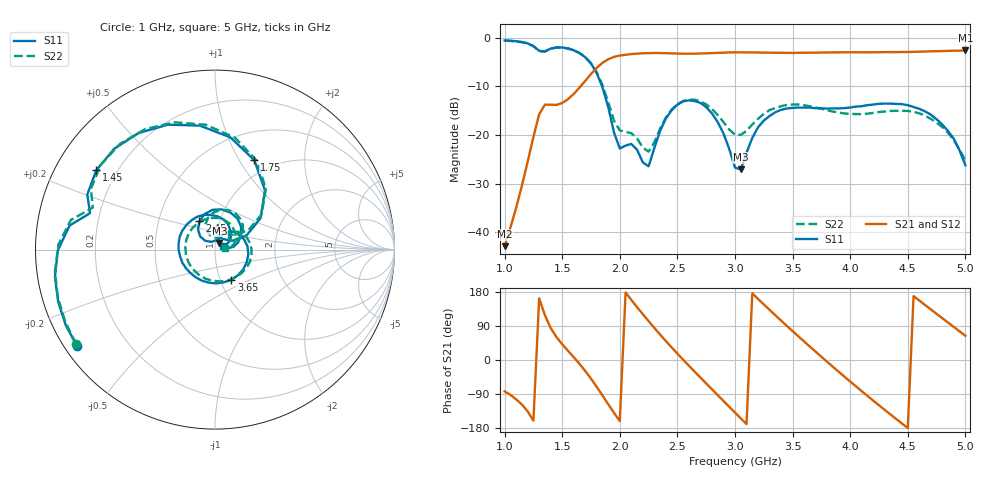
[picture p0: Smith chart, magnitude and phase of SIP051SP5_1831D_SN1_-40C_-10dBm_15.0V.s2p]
# GHz  S  dB  R  50
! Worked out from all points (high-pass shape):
!   81 points, 1 GHz to 5 GHz, reference 50 ohm
!   highest |S21| = -2.62 dB at 5 GHz (marker M1); lowest = -42.8 dB at 1 GHz (marker M2)
!   |S21| within 3 dB of the highest: 1.827 GHz to end of sweep
!   lowest |S11| = -27.1 dB at 3.05 GHz (marker M3), VSWR 1.09, Z = 52.4 + j3.84 ohm
!   |S11| at or under -10 dB: 1.846 GHz to end of sweep
!   |S22| runs from -25.2 to -0.6 dB; largest |S21 - S12| = 0.0022
!   S11 on the Smith chart (normalised r, x): 1 GHz: 0.03, -0.31; 1.45 GHz: 0.12, +0.30; 1.75 GHz: 0.82, +1.16; 2.45 GHz: 0.80, +0.26; 3.65 GHz: 1.13, -0.39; 5 GHz: 1.09, +0.05
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1  -0.55 -145.0  -42.85 -82.8  -43.25 -83.3  -0.58 -145.8
1.3  -2.68 164.6  -15.73 162.6  -15.70 162.4  -2.73 162.0
1.45  -1.99 146.2  -13.80 60.6  -13.80 60.5  -2.02 143.3
1.7  -4.00 82.1  -8.86 -28.9  -8.86 -28.9  -3.97 79.9
1.75  -5.29 66.2  -7.45 -49.3  -7.44 -49.3  -5.24 64.8
1.9  -14.29 24.2  -4.42 -116.9  -4.41 -116.8  -13.28 30.3
2.05  -22.17 74.4  -3.50 178.2  -3.49 178.4  -19.35 60.5
2.25  -26.43 115.5  -3.16 102.6  -3.15 102.6  -23.41 89.7
2.35  -19.11 138.5  -3.14 67.1  -3.13 67.1  -18.66 114.3
2.45  -14.90 119.0  -3.21 33.3  -3.20 33.2  -14.76 101.8
2.75  -14.26 41.5  -3.20 -61.9  -3.19 -61.8  -13.70 41.1
3  -26.70 21.0  -3.00 -138.9  -2.99 -138.8  -19.92 30.8
3.05  -27.08 55.7  -2.99 -153.9  -2.99 -154.0  -19.98 39.7
3.2  -18.40 56.1  -3.03 161.2  -3.03 161.2  -16.68 42.5
3.4  -14.81 6.0  -3.09 104.0  -3.08 103.9  -14.06 10.6
3.65  -14.36 -61.5  -3.06 35.3  -3.06 35.3  -14.08 -42.2
3.7  -14.47 -74.8  -3.06 21.9  -3.05 21.9  -14.35 -54.8
4.05  -14.15 -158.2  -2.98 -69.5  -2.98 -69.6  -15.68 -153.9
4.35  -13.54 138.5  -2.94 -143.8  -2.96 -143.8  -15.04 120.8
4.6  -14.61 85.8  -2.86 156.9  -2.86 156.8  -15.53 61.4
4.8  -17.84 46.3  -2.74 110.2  -2.73 110.2  -18.35 22.1
5  -26.20 24.9  -2.62 63.9  -2.62 63.9  -25.24 7.7
